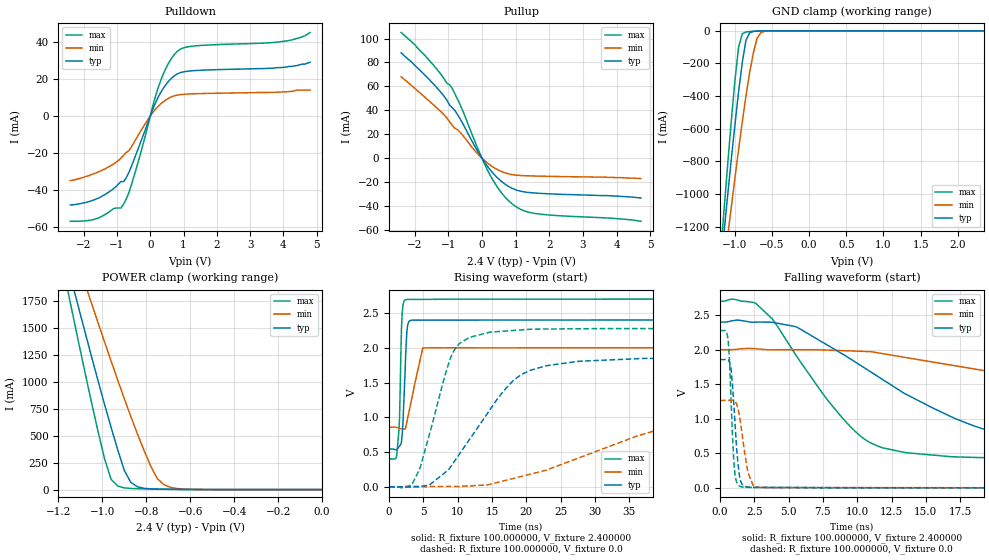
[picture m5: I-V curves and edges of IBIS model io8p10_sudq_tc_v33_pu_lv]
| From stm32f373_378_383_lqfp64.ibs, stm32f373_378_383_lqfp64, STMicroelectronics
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|   Model io8p10_sudq_tc_v33_pu_lv
[Model]  io8p10_sudq_tc_v33_pu_lv
Model_type I/O
Polarity   Non-Inverting
Enable   Active-Low
Vinl =   0.720000V
Vinh =   1.680000V
Vmeas =  1.200000V
Cref =   50.000000pF
Rref =   100.000000M
Vref =   0.0V
C_comp   1.373400pF   1.288200pF   1.481900pF
[Temperature Range]   25.000000   0.125000k   -40.000000
[Pullup Reference]   2.400000V   2.000000V   2.700000V
[Pulldown Reference]   0.0V   0.0V   0.0V
[POWER Clamp Reference]   2.400000V   2.000000V   2.700000V
[GND Clamp Reference]   0.0V   0.0V   0.0V
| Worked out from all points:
|   slope of the pulldown table from 0 to 0.36 V, typ, clamps not added: 25.7 ohm
|   slope of the pullup table from 0 to 0.36 V, typ, clamps not added: 26.8 ohm
|   GND clamp passes 1 mA (typ) near -0.67 V on its own axis
|   POWER clamp passes 1 mA (typ) near -0.60 V on its own axis
|   rising waveform, R_fixture 100.000000, V_fixture 2.400000: 20-80 % time 461ps typ, 1.48ns min, 342ps max; typ from 0.543 V to 2.4 V
|   rising waveform, R_fixture 100.000000, V_fixture 0.0: 20-80 % time 8.11ns typ, 22.7ns min, 3.8ns max; typ from 0.001 V to 1.86 V
|   falling waveform, R_fixture 100.000000, V_fixture 2.400000: 20-80 % time 10.1ns typ, 23.6ns min, 5.13ns max; typ from 2.4 V to 0.543 V
|   falling waveform, R_fixture 100.000000, V_fixture 0.0: 20-80 % time 392ps typ, 570ps min, 290ps max; typ from 1.86 V to 0.001 V
[Pulldown]
|Voltage   I(typ)   I(min)   I(max)
-2.4V     -47.9mA    -34.8mA    -56.7mA
-1.6V     -44.5mA    -30.4mA    -55.2mA
-880mV    -35.33mA   -22.63mA   -49.55mA
-800mV    -35.33mA   -21.13mA   -47.42mA
-640mV    -30.33mA   -18.65mA   -41.16mA
-480mV    -23.12mA   -14mA      -31.94mA
240mV     10.22mA    5.339mA    15.38mA
480mV     17.22mA    8.864mA    26.1mA
800mV     22.59mA    11.27mA    34.68mA
1.28V     24.44mA    12mA       37.7mA
4.16V     26.7mA     13.2mA     40.7mA
4.8V      29mA       14mA       45mA
[Pullup]
|Voltage   I(typ)   I(min)   I(max)
-2.4V     88mA       68mA       105mA
-2V       77.8mA     58.5mA     95mA
-1.36V    59.6mA     42.5mA     75.1mA
-880mV    42.12mA    27.44mA    58.22mA
-560mV    28.45mA    18.75mA    39mA
-160mV    7.44mA     4.66mA     10.64mA
160mV     -6.607mA   -3.947mA   -9.704mA
480mV     -16.91mA   -9.806mA   -25.1mA
880mV     -24.89mA   -13.63mA   -37.75mA
1.2V      -27.87mA   -14.5mA    -43.37mA
1.6V      -29.13mA   -14.89mA   -46.24mA
4.72V     -33.2mA    -17mA      -52.7mA
[GND_clamp]
|Voltage   I(typ)   I(min)   I(max)
-2.4V     -7.358A    -6.372A    -8.78A
-1.2V     -1.489A    -1.65A     -1.416A
-1.15V    -1.254A    -1.461A    -1.124A
-1.1V     -1.024A    -1.273A    -838.2mA
-1.05V    -797.6mA   -1.088A    -563.1mA
-950mV    -374.6mA   -728.7mA   -100.8mA
-900mV    -194.3mA   -557.9mA   -18.01mA
-850mV    -56.94mA   -397.4mA   -7.08mA
-750mV    -3.582mA   -133.8mA   -2.771mA
-700mV    -1.516mA   -44.7mA    -1.516mA
-600mV    -235.4uA   -2.939mA   -209.5uA
2.35V     0A         0A         0A
[POWER_clamp]
|Voltage   I(typ)   I(min)   I(max)
-2.4V     9.979A     9.967A     9.901A
-1.17V    2.182A     2.481A     1.978A
-1.14V    1.945A     2.294A     1.683A
-1.11V    1.71A      2.108A     1.391A
-1.08V    1.476A     1.923A     1.102A
-1.05V    1.245A     1.739A     819.9mA
-960mV    578.3mA    1.196A     96.08mA
-900mV    179.5mA    846.7mA    16.05mA
-870mV    67.19mA    678.8mA    10.83mA
-780mV    6.763mA    219.9mA    5.868mA
-720mV    3.368mA    46.35mA    3.823mA
0V        0A         0A         0A
[Ramp]
| variable   typ   min   max
dV/dt_r  1.11273/8.10567n   0.75768/22.67004n   1.36520/3.79452n
dV/dt_f  1.11401/10.12196n   0.68578/23.64273n   1.37909/5.12498n
R_load = 100.000000
[Rising Waveform]
R_fixture= 100.000000
V_fixture= 2.400000
V_fixture_min= 2.000000
V_fixture_max= 2.700000
|time   V(typ)   V(min)   V(max)
0s        543.1mV    857mV      401.7mV
1.101ns   531.6mV    855.1mV    451.4mV
1.502ns   584.8mV    841.1mV    954.7mV
1.802ns   651mV      834.5mV    2.296V
1.902ns   758.5mV    833.6mV    2.503V
2.402ns   1.877V     845.4mV    2.692V
2.603ns   2.256V     940.8mV    2.696V
2.803ns   2.363V     1.036V     2.697V
4.905ns   2.398V     1.998V     2.696V
49.85ns   2.4V       2V         2.7V
[Rising Waveform]
R_fixture= 100.000000
V_fixture= 0.0
V_fixture_min= 0.0
V_fixture_max= 0.0
|time   V(typ)   V(min)   V(max)
0s        956.5uV    1.197mV    860.5uV
3.203ns   2.702mV    -815.7uV   27.1mV
4.404ns   4.791mV    -1.364mV   246.6mV
9.409ns   352.3mV    4.583mV    1.956V
14.61ns   1.099V     34.4mV     2.224V
19.42ns   1.622V     153.7mV    2.259V
27.63ns   1.806V     415.4mV    2.274V
45.65ns   1.852V     1.007V     2.276V
53.45ns   1.856V     1.139V     2.276V
99.7ns    1.856V     1.267V     2.276V
[Falling Waveform]
R_fixture= 100.000000
V_fixture= 2.400000
V_fixture_min= 2.000000
V_fixture_max= 2.700000
|time   V(typ)   V(min)   V(max)
0s        2.4V       2V         2.7V
2.603ns   2.399V     2.014V     2.672V
5.606ns   2.327V     2V         1.899V
9.61ns    1.853V     1.981V     865.6mV
11.01ns   1.675V     1.971V     647.3mV
13.61ns   1.349V     1.884V     509mV
20.62ns   772.3mV    1.647V     429.8mV
29.83ns   595.5mV    1.322V     407.4mV
57.26ns   543.3mV    917.9mV    401.9mV
99.7ns    543.1mV    857mV      401.7mV
[Falling Waveform]
R_fixture= 100.000000
V_fixture= 0.0
V_fixture_min= 0.0
V_fixture_max= 0.0
|time   V(typ)   V(min)   V(max)
0s        1.856V     1.267V     2.276V
600.6ps   1.852V     1.268V     2.135V
800.8ps   1.734V     1.271V     1.298V
1.001ns   1.241V     1.266V     407.4mV
1.101ns   913.1mV    1.252V     170.8mV
1.401ns   197.7mV    1.066V     27.9mV
1.602ns   55.26mV    793.3mV    13.53mV
2.102ns   9.396mV    190.4mV    8.458mV
2.903ns   6.351mV    8.615mV    8.412mV
49.85ns   956.5uV    1.197mV    860.5uV
